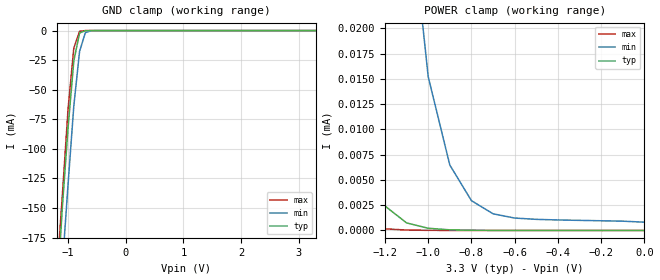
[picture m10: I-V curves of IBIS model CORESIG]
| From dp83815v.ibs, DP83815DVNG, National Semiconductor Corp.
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|   Model CORESIG
[Model]   CORESIG
Model_type   Input
Vinl =   0.80V
Vinh =   2.00V
Vmeas =   1.50V
Cref =  10.00pF
Rref =  50.00
C_comp   4.00pF   4.00pF   4.00pF
[Temperature Range]   27.00   100.00   0.000
[Voltage Range]   3.30V   3.00V   3.60V
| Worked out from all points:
|   GND clamp passes 1 mA (typ) near -0.75 V on its own axis
|   POWER clamp passes 1 mA (typ) near -1.98 V on its own axis
[GND_clamp]
| voltage   I(typ)   I(min)   I(max)
-3.3V     -1.95A     -1.99A     -1.93A
-1.2V     -230mA     -270mA     -210mA
-1.1V     -150mA     -200mA     -140mA
-1V       -82.13mA   -130mA     -66.23mA
-900mV    -25.64mA   -63.58mA   -14.7mA
-800mV    -2.04mA    -17.56mA   -590uA
-700mV    -65.88uA   -1.76mA    -12.72uA
-600mV    -1.97uA    -110uA     -270nA
3.3V      9.66pA     1uA        3.07pA
[POWER_clamp]
| voltage   I(typ)   I(min)   I(max)
-3.3V     160mA      350mA      68.04mA
-1.6V     130uA      720uA      19.61uA
-1.5V     54.22uA    470uA      6.52uA
-1.4V     20.71uA    280uA      2.04uA
-1.3V     7.3uA      160uA      590nA
-1.2V     2.42uA     77.68uA    160nA
-1.1V     750nA      35.4uA     42.11nA
-1V       220nA      15.21uA    12.91nA
-900mV    62.61nA    6.47uA     6.04nA
-800mV    19.86nA    2.95uA     4.19nA
-600mV    5.62nA     1.23uA     2.1nA
0V        9.66pA     820nA      3.71pA
